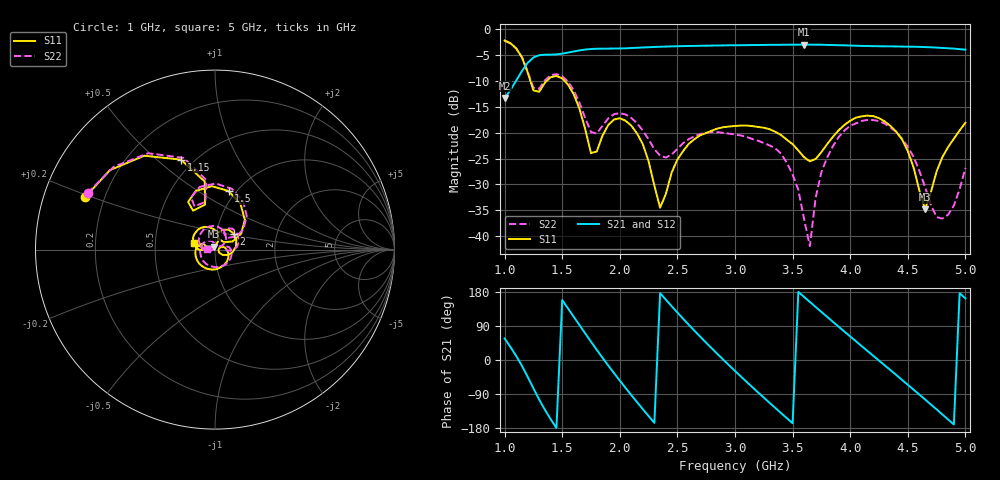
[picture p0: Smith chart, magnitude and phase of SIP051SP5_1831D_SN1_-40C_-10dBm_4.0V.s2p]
# GHz  S  dB  R  50
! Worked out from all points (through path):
!   81 points, 1 GHz to 5 GHz, reference 50 ohm
!   highest |S21| = -2.97 dB at 3.6 GHz (marker M1); lowest = -13.3 dB at 1 GHz (marker M2)
!   lowest |S11| = -34.8 dB at 4.65 GHz (marker M3), VSWR 1.04, Z = 49.3 + j1.66 ohm
!   |S11| at or under -10 dB: 1.224 GHz to 1.365 GHz (141.2 MHz wide, 10.9 % of centre); 1.521 GHz to end of sweep
!   |S22| runs from -41.9 to -2.2 dB; largest |S21 - S12| = 0.0023
!   S11 on the Smith chart (normalised r, x): 1 GHz: 0.13, +0.19; 1.15 GHz: 0.43, +0.60; 1.5 GHz: 0.92, +0.68; 2 GHz: 1.22, +0.22; 5 GHz: 0.78, +0.06
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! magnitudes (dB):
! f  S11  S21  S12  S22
! 1 GHz  -2.2  -13.3  -13.3  -2.2
! 1.15 GHz  -5.4  -8.1  -8.1  -5.4
! 1.25 GHz  -11.8  -5.4  -5.5  -11.3
! 1.5 GHz  -9.5  -4.7  -4.7  -9.1
! 1.7 GHz  -19.3  -3.9  -3.9  -17.2
! 1.8 GHz  -23.6  -3.8  -3.8  -20.2
! 2 GHz  -17.2  -3.7  -3.7  -16.2
! 2.2 GHz  -22.2  -3.5  -3.5  -19.6
! 2.35 GHz  -34.5  -3.4  -3.4  -24.4
! 2.6 GHz  -22.1  -3.2  -3.2  -21.2
! 3 GHz  -18.7  -3.1  -3.1  -20.3
! 3.4 GHz  -20.5  -3.0  -3.0  -24.1
! 3.6 GHz  -24.7  -3.0  -3.0  -36.7
! 3.65 GHz  -25.5  -3.0  -3.0  -41.9
! 3.7 GHz  -25.1  -3.0  -3.0  -32.6
! 3.8 GHz  -22.2  -3.0  -3.0  -24.8
! 3.95 GHz  -18.5  -3.1  -3.1  -19.6
! 4.35 GHz  -18.7  -3.3  -3.3  -19.0
! 4.5 GHz  -23.6  -3.4  -3.4  -22.7
! 4.65 GHz  -34.8  -3.4  -3.4  -30.5
! 4.8 GHz  -24.7  -3.6  -3.6  -36.6
! 5 GHz  -18.1  -3.9  -3.9  -26.8
